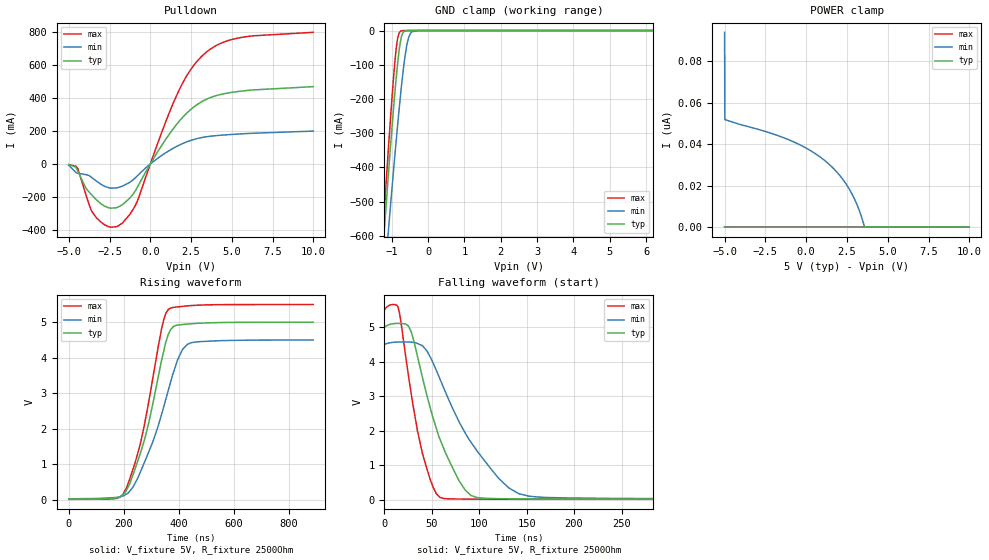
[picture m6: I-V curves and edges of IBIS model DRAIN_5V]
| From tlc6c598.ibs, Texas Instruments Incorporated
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|   Model DRAIN_5V
[Model]   DRAIN_5V
Model_type   Open_drain
Polarity   Non-Inverting
Vmeas = 2.25
Vref = 5
Cref = 15pF
Rref = 2500
|   typ   min   max
|   (nom PVT)   (fast PVT)   (slow PVT)
C_comp   1.348p   1.226p   1.507p
|C_comp (Hi state)   2.095p   1.738p   2.284p
|C_comp (Low state)   3.024p   2.164p   3.482p
[Voltage Range]   5   4.5   5.5
[Temperature Range]   27   150   -40
[Pullup Reference]   5   4.5   5.5
[Pulldown Reference]   -0   -0   -0
[Power Clamp Reference]   5   4.5   5.5
[GND Clamp Reference]   -0   -0   -0
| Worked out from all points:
|   slope of the pulldown table from 0 to 0.75 V, typ, clamps not added: 6.25 ohm
|   GND clamp passes 1 mA (typ) near -0.62 V on its own axis
|   falling waveform, V_fixture 5V, R_fixture 2500Ohm: 20-80 % time 34.2ns typ, 54.6ns min, 21.4ns max; typ from 5 V to 0.012 V
|   rising waveform, V_fixture 5V, R_fixture 2500Ohm: 20-80 % time 92.5ns typ, 113ns min, 84.1ns max; typ from 0.012 V to 5 V
[Pulldown]
|   Voltage   I(typ)   I(min)   I(max)
-5V       -3.582mA   -7.974mA   -3.896mA
-4.445V   -43.22mA   -55.56mA   -28.55mA
-3.605V   -185.9mA   -80.75mA   -283.8mA
-3.305V   -216.9mA   -103.6mA   -325.1mA
-2.6V     -263.3mA   -142.2mA   -377mA
-1.97V    -260.3mA   -142.5mA   -374.7mA
-905mV    -159.8mA   -82.07mA   -248.1mA
1.615V    239.6mA    106.2mA    415mA
2.26V     309.9mA    134.6mA    537.5mA
3.085V    372.6mA    158.4mA    644.3mA
5.185V    435.4mA    179.7mA    756.8mA
9.985V    467.4mA    198.8mA    795.6mA
[GND Clamp]
|   Voltage   I(typ)   I(min)   I(max)
-5V       -6.964A    -6.265A    -7.581A
-1.25V    -651.7mA   -792.7mA   -598.5mA
-1.085V   -411.3mA   -577.9mA   -335.3mA
-950mV    -228.3mA   -409.4mA   -138.4mA
-875mV    -137mA     -319.9mA   -51.72mA
-830mV    -88.93mA   -268.1mA   -19.62mA
-740mV    -21.63mA   -170.8mA   -1.294mA
-650mV    -2.008mA   -87.42mA   -66.98uA
-530mV    -35.81uA   -19.01mA   -1.15uA
-440mV    -1.495uA   -3.406mA   0A
-275mV    0A         -68.47uA   0A
9.985V    0A         0A         0A
[POWER Clamp]
|   Voltage   I(typ)   I(min)   I(max)
-5V       154.6pA    93.92nA    161.5pA
-4.985V   77.32pA    51.84nA    80.74pA
-1.25V    0A         42.72nA    0A
-20mV     0A         38.19nA    0A
985mV     0A         33.06nA    0A
1.825V    0A         27.05nA    0A
2.545V    0A         19.6nA     0A
2.86V     0A         15.21nA    0A
3.085V    0A         11.41nA    0A
3.295V    0A         7.187nA    0A
3.595V    0A         0A         0A
9.985V    0A         0A         0A
[Ramp]
R_load = 2500
|   typ   min   max
dV/dt_r   2.99283/9.2495e-08   2.68605/1.13494e-07   3.29531/8.40556e-08
dV/dt_f   2.99287/3.42288e-08   2.68621/5.46257e-08   3.29532/2.13633e-08
[Falling Waveform]
V_fixture = 5V
V_fixture_min = 4.5V
V_fixture_max = 5.5V
R_fixture = 2500Ohm
C_fixture = 0F
|   Time   V(typ)   V(min)   V(max)
0s        5V         4.5V       5.5V
14.28ns   5.11V      4.569V     5.585V
25.23ns   5.035V     4.569V     3.613V
40.05ns   3.546V     4.463V     1.339V
51.62ns   2.338V     3.941V     339.6mV
62.65ns   1.475V     3.229V     31.68mV
91.21ns   119.8mV    1.665V     12.85mV
131.2ns   23.61mV    336.9mV    10.27mV
152.4ns   18.98mV    99.75mV    9.444mV
890ns     11.89mV    22.76mV    7.801mV
[Rising Waveform]
V_fixture = 5V
V_fixture_min = 4.5V
V_fixture_max = 5.5V
R_fixture = 2500Ohm
C_fixture = 0F
|   Time   V(typ)   V(min)   V(max)
0s        11.86mV    22.53mV    7.798mV
178.7ns   53.67mV    69.21mV    37.48mV
209.6ns   260.5mV    153.5mV    323.6mV
248.2ns   1.019V     561mV      1.215V
277.8ns   1.743V     1.093V     2.208V
338.3ns   3.936V     2.411V     4.829V
363ns     4.668V     3.1V       5.364V
414.1ns   4.935V     4.232V     5.448V
444.5ns   4.956V     4.42V      5.469V
890ns     5V         4.499V     5.5V
